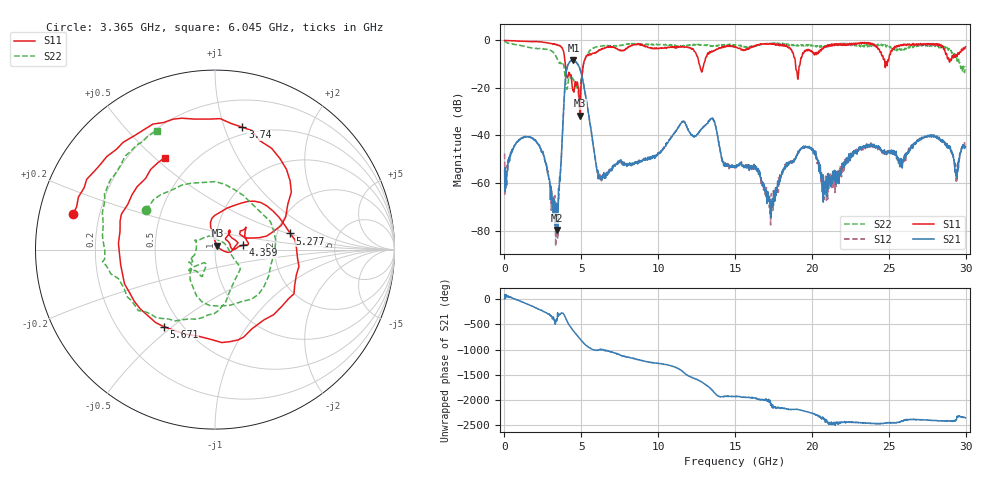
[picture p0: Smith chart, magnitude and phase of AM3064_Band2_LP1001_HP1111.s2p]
# Hz S DB R 50.0
!freq dBS11 angS11 dBS21 angS21 dBS12 angS12 dBS22 angS22
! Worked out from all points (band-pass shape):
!   1600 points, 10 MHz to 29.98 GHz, reference 50 ohm
!   highest |S21| = -8.33 dB at 4.49 GHz (marker M1); lowest = -79.7 dB at 3.403 GHz (marker M2)
!   |S21| within 3 dB of the highest: 4.081 GHz to 4.871 GHz (789.8 MHz wide, 17.6 % of centre)
!   lowest |S11| = -31.7 dB at 4.921 GHz (marker M3), VSWR 1.05, Z = 51.3 + j2.29 ohm
!   |S11| at or under -10 dB: 3.957 GHz to 5.139 GHz (1.182 GHz wide, 26 % of centre); 12.67 GHz to 12.96 GHz (288.3 MHz wide, 2.25 % of centre); 18.93 GHz to 19.23 GHz (293.9 MHz wide, 1.54 % of centre)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
!   |S22| runs from -24.9 to -0.3 dB; largest |S21 - S12| = 0.011
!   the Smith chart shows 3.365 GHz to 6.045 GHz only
!   S11 on the Smith chart (normalised r, x): 3.365 GHz: 0.10, +0.12; 3.74 GHz: 0.43, +1.15; 4.359 GHz: 1.36, +0.07; 5.277 GHz: 2.36, +0.52; 5.671 GHz: 0.40, -0.47; 6.045 GHz: 0.35, +0.54
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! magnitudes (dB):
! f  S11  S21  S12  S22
! 10 MHz  -0.1  -54.6  -47.6  -0.3
! 1.866 GHz  -0.6  -41.2  -41.4  -3.3
! 3.365 GHz  -1.8  -68.6  -68.4  -7.1
! 3.403 GHz  -1.8  -79.7  -73.7  -7.3
! 3.74 GHz  -3.1  -44.0  -43.6  -9.2
! 4.021 GHz  -14.3  -13.3  -13.5  -20.2
! 4.359 GHz  -16.1  -8.6  -8.4  -15.4
! 4.49 GHz  -21.3  -8.3  -8.5  -17.0
! 4.921 GHz  -31.7  -12.2  -12.2  -22.3
! 5.015 GHz  -16.3  -14.4  -14.2  -15.0
! 5.277 GHz  -7.4  -23.2  -23.1  -7.2
! 5.671 GHz  -5.8  -39.6  -39.4  -3.9
! 6.045 GHz  -4.7  -54.3  -55.7  -2.7
! 10 GHz  -3.4  -47.8  -47.2  -1.8
! 13.49 GHz  -4.5  -32.9  -32.8  -2.3
! 15 GHz  -2.5  -53.3  -53.2  -1.9
! 17.37 GHz  -1.5  -70.7  -64.4  -1.2
! 19.99 GHz  -4.5  -46.0  -45.4  -1.9
! 20.87 GHz  -2.5  -59.0  -58.4  -2.9
! 25 GHz  -8.1  -46.7  -46.3  -2.3
! 29.38 GHz  -6.0  -57.0  -59.2  -7.1
! 29.98 GHz  -2.7  -44.7  -44.7  -10.9
